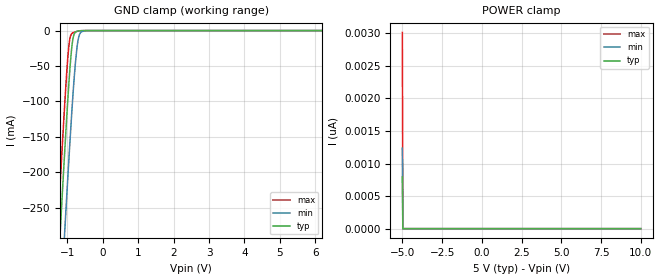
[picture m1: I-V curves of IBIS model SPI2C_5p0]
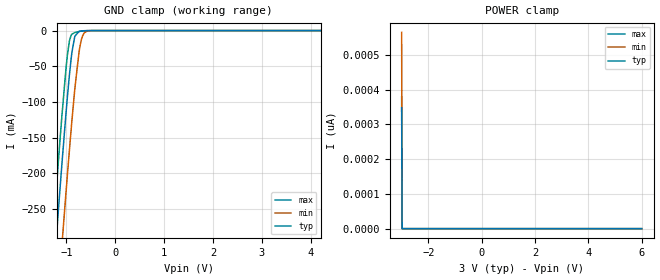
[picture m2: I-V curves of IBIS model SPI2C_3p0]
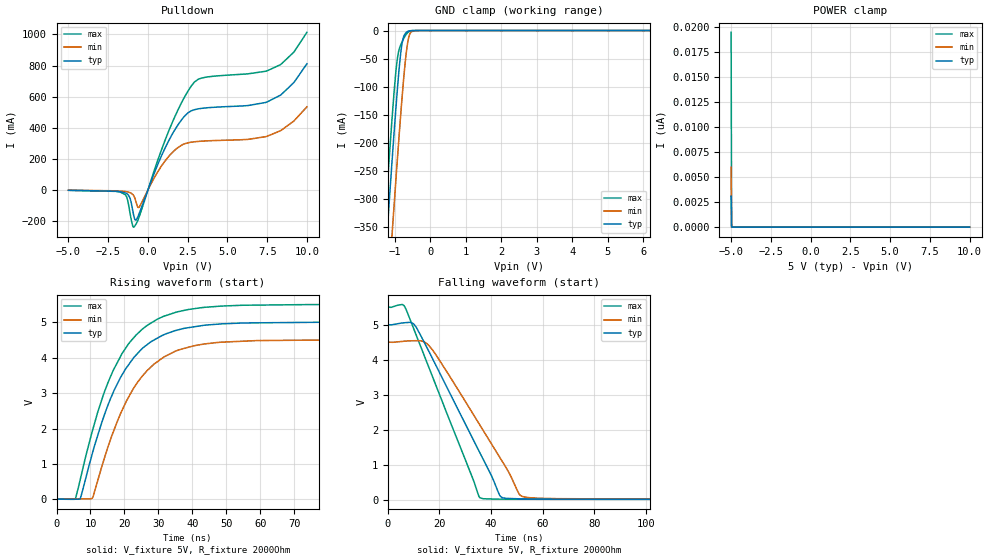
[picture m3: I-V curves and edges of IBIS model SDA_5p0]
|Texas Instruments Incorporated
|  part#   Digital Voltage Range
| DACx0501   2.7V - 5.5V
[IBIS Ver]   4.1
[File name]   dacx0501.ibs
[File Rev]   1.0
[Date]   01/11/2019
[Source]
| Texas Instruments Incorporated.
| 12500 TI Blvd
| Dallas, TX -75243
[Notes]   Revision History:
| Rev 1.0: 01/11/2019
| - Initial version of the model
| - Model generated from simulations in TISPICE
| - C_comp although listed in numerical order of value are
|   obtained from varying PVT conditions. For PVT conditions for
|   each specific value refer the buffer description under
|   respective [Model]. IBIS model user is responsible for using
|   appropriate C_comp to simulate for Signal Integrity.
| - Warnings regarding combined Non-monotonicity of various models have been
|   reviewed and considered minor and can be ignored.
| - Model names with a trailing _3p0 contain the model for
|   3.0V operation. Model names with a trailing _5p0 contain the model
|   for 5.0V operation.
[Disclaimer]
| This model is designed as an aid for customers of Texas Instruments.
| TI and its licensors and suppliers make no warranties, either expressed
| or implied, with respect to this  model, including the warranties of
| merchantability or fitness for a particular purpose. The model is
| provided solely on an "as is" basis. The entire risk as to its quality
| and performance is with the customer.
| This model is subject to change without notice. Texas Instruments
| Incorporated is not responsible for updating this model.
[Copyright]
 (C) Copyright 2019 Texas Instruments Incorporated. All rights reserved.
|   Device
[Component]  DACX0501DQF | 8 pin VSON
[Manufacturer]   TI
[Package]
| variable   typ   min   max
R_pkg   0.05   0.04   0.06
L_pkg   1.0nH   0.8nH   1.2nH
C_pkg   0.2pF   0.16pF   0.24pF
[Pin]  signal_name   model_name   R_pin   L_pin   C_pin
1   VDD   POWER   na   na   na
2   VOUT   NC   na   na   na
3   AGND   GND   na   na   na
4   SPI2C   SPI2C   na   na   na
5   SCLK/SCL   SCL   na   na   na
6   SYNCB/A0   SCL   na   na   na
7   SDIN/SDA   SDA   na   na   na
8   VREFIO   NC   na   na   na
[Component]  DACX0501DGS | 10 pin MSOP
[Manufacturer]   TI
[Package]
| variable   typ   min   max
R_pkg   0.05   0.04   0.06
L_pkg   1.0nH   0.8nH   1.2nH
C_pkg   0.2pF   0.16pF   0.24pF
[Pin]  signal_name   model_name   R_pin   L_pin   C_pin
1   VDD   POWER   na   na   na
2   VOUT   NC   na   na   na
3   NC   NC   na   na   na
4   AGND   GND   na   na   na
5   SPI2C   SPI2C   na   na   na
6   SCLK/SCL   SCL   na   na   na
7   SYNCB/A0   SCL   na   na   na
8   SDIN/SDA   SDA   na   na   na
9   NC   NC   na   na   na
10   VREFIO   NC   na   na   na
|   Model Selectors
[Model Selector]  SDA
SDA_3p0  I/O open drain buffer at 3.0V operation
SDA_5p0  I/O open drain buffer at 5.0V operation
[Model Selector]  SCL
SCL_3p0   input buffer at 3.0V operation
SCL_5p0   input buffer at 5.0V operation
[Model Selector]  SPI2C
SPI2C_3p0   input buffer at 3.0V operation
SPI2C_5p0   input buffer at 5.0V operation
| Models and submodels in the file (6): SPI2C_5p0 (Input), SPI2C_3p0 (Input), SDA_5p0 (I/O_open_drain), SDA_3p0 (I/O_open_drain), SCL_5p0 (Input), SCL_3p0 (Input)
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|   Model
[Model]   SPI2C_5p0
Model_type   Input
Vinl = 1.5
Vinh = 3.5
|   typ   min   max
C_comp   0.423pF   0.377pF   0.481pF
[Voltage Range]   5   4.5   5.5
[Temperature Range]   25   125   -40
[Power Clamp Reference]   5   4.5   5.5
[GND Clamp Reference]   0   0   0
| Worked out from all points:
|   GND clamp passes 1 mA (typ) near -0.73 V on its own axis
[GND Clamp]
|   Voltage   I(typ)   I(min)   I(max)
-5V       -4.018A    -4.121A    -3.958A
-1.43V    -501.2mA   -615.9mA   -432.8mA
-1.25V    -331.9mA   -447mA     -263mA
-1.16V    -249.3mA   -364.1mA   -180.8mA
-1.085V   -182.4mA   -296.2mA   -115.2mA
-1.04V    -143.7mA   -256.2mA   -78.36mA
-950mV    -71.94mA   -178.6mA   -19.98mA
-875mV    -25.31mA   -118mA     -4.433mA
-800mV    -4.408mA   -64.17mA   -2.261mA
-680mV    -446.2uA   -10.05mA   -678.1uA
-500mV    -9.097uA   -173.1uA   -17.18uA
10V       0A         0A         0A
[POWER Clamp]
|   Voltage   I(typ)   I(min)   I(max)
-5V       793pA      1.236nA    3.013nA
-4.97V    0A         0A         0A
-4.955V   0A         0A         0A
10V       0A         0A         0A
|   Model
[Model]   SPI2C_3p0
Model_type   Input
Vinl = 0.9
Vinh = 2.1
|   typ   min   max
C_comp   0.423pF   0.377pF   0.481pF
[Voltage Range]   3   2.7   3.3
[Temperature Range]   25   125   -40
[Power Clamp Reference]   3   2.7   3.3
[GND Clamp Reference]   0   0   0
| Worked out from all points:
|   GND clamp passes 1 mA (typ) near -0.73 V on its own axis
[GND Clamp]
|   Voltage   I(typ)   I(min)   I(max)
-3V       -2.035A    -2.143A    -1.972A
-1.281V   -360.7mA   -475.8mA   -291.9mA
-1.146V   -236.7mA   -351.3mA   -168.2mA
-1.092V   -188.6mA   -302.4mA   -121.1mA
-1.011V   -119.5mA   -230.8mA   -56.49mA
-939mV    -64.04mA   -169.5mA   -15.61mA
-885mV    -30.31mA   -125.8mA   -5.092mA
-831mV    -9.604mA   -85.27mA   -2.895mA
-705mV    -676.1uA   -16.7mA    -909.7uA
-642mV    -228.2uA   -4.238mA   -403.6uA
-552mV    -33.57uA   -536.7uA   -69.65uA
6V        0A         0A         0A
[POWER Clamp]
|   Voltage   I(typ)   I(min)   I(max)
-3V       347.9pA    564.7pA    379.3pA
-2.982V   0A         0A         0A
-2.973V   0A         0A         0A
6V        0A         0A         0A
|   Model
[Model]   SDA_5p0
Model_type   I/O_open_drain
Polarity   Non-Inverting
Enable   Active-Low
Vinl = 1.5
Vinh = 3.5
Vmeas = 2.5
Vref = 5
Cref = 1pF
Rref = 2000
|   typ   min   max
C_comp   3.377pF   3.057pF   3.504pF
[Voltage Range]   5   4.5   5.5
[Temperature Range]   25   125   -40
[Pullup Reference]   5   4.5   5.5
[Pulldown Reference]   0   0   0
[Power Clamp Reference]   5   4.5   5.5
[GND Clamp Reference]   0   0   0
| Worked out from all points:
|   slope of the pulldown table from 0 to 0.75 V, typ, clamps not added: 3.83 ohm
|   GND clamp passes 1 mA (typ) near -0.61 V on its own axis
|   falling waveform, V_fixture 5V, R_fixture 2000Ohm: 20-80 % time 20.5ns typ, 22.6ns min, 17.6ns max; typ from 5 V to 0.009 V
|   rising waveform, V_fixture 5V, R_fixture 2000Ohm: 20-80 % time 13ns typ, 13.1ns min, 13ns max; typ from 0.009 V to 5 V
[Pulldown]
|   Voltage   I(typ)   I(min)   I(max)
-5V       -2.015mA   -1.612mA   -2.004mA
-1.415V   -18.81mA   -10.03mA   -30.58mA
-1.13V    -51.47mA   -17.01mA   -147.1mA
-875mV    -172.4mA   -40.36mA   -237.7mA
-755mV    -193.7mA   -74.64mA   -220.1mA
-560mV    -153.6mA   -110.9mA   -175.3mA
1.36V     327.1mA    222.1mA    392.2mA
2.245V    467.7mA    294.4mA    586.7mA
2.905V    515.7mA    309.7mA    691.5mA
7.495V    565.8mA    345.4mA    766.1mA
9.16V     688.7mA    441.9mA    884.5mA
10V       811.4mA    534.7mA    1.014A
[GND Clamp]
|   Voltage   I(typ)   I(min)   I(max)
-5V       -4.075A    -4.197A    -4.003A
-1.43V    -557mA     -689.3mA   -477.9mA
-1.25V    -386.7mA   -519.1mA   -307.9mA
-1.145V   -289.5mA   -421.3mA   -211.9mA
-1.085V   -235.2mA   -366.1mA   -159.4mA
-1.055V   -208.5mA   -338.8mA   -134.2mA
-950mV    -119.3mA   -245mA     -59.1mA
-830mV    -36.45mA   -143.6mA   -24.41mA
-710mV    -5.467mA   -56.39mA   -9.431mA
-620mV    -1.144mA   -14.6mA    -2.617mA
-410mV    -5.32uA    -78.75uA   -6.596uA
10V       0A         0A         0A
[POWER Clamp]
|   Voltage   I(typ)   I(min)   I(max)
-5V       3.107nA    5.988nA    19.48nA
-4.97V    0A         0A         0A
-4.955V   0A         0A         0A
10V       0A         0A         0A
[Ramp]
R_load = 2000
|   typ   min   max
dV/dt_r   2.99475/1.30305e-08   2.69358/1.3102e-08   3.29494/1.2999e-08
dV/dt_f   2.99475/2.04384e-08   2.69358/2.2555e-08   3.29494/1.7592e-08
[Falling Waveform]
V_fixture = 5V
V_fixture_min = 4.5V
V_fixture_max = 5.5V
R_fixture = 2000Ohm
C_fixture = 0F
|   Time   V(typ)   V(min)   V(max)
0s        5V         4.5V       5.5V
6.136ns   5.052V     4.525V     5.553V
10.8ns    4.945V     4.542V     4.735V
17.22ns   4.04V      4.285V     3.528V
35.25ns   1.399V     2.18V      103mV
36.76ns   1.178V     1.998V     28.07mV
44.02ns   68.39mV    1.13V      13.14mV
51.06ns   23.02mV    142.5mV    11.9mV
58.2ns    16.32mV    39.32mV    10.64mV
500ns     8.749mV    10.7mV     8.432mV
[Rising Waveform]
V_fixture = 5V
V_fixture_min = 4.5V
V_fixture_max = 5.5V
R_fixture = 2000Ohm
C_fixture = 0F
|   Time   V(typ)   V(min)   V(max)
0s        8.748mV    10.7mV     8.432mV
5.572ns   7.709mV    14.02mV    22.36mV
7.02ns    34.77mV    14.88mV    578mV
10.59ns   1.312V     44.51mV    1.945V
15.25ns   2.689V     1.515V     3.322V
21.07ns   3.78V      2.862V     4.371V
28.63ns   4.495V     3.812V     5.024V
42.56ns   4.901V     4.371V     5.41V
79.62ns   4.999V     4.499V     5.498V
500ns     5V         4.5V       5.5V
